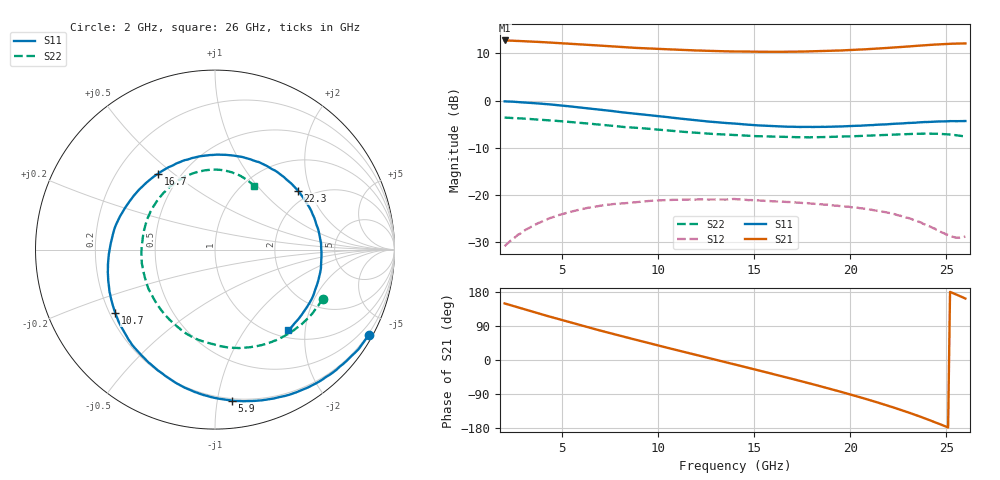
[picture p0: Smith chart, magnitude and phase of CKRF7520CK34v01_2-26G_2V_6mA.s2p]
! CHUO DENSHI KOGYO Co.,Ltd.
! 1. March 2016
! CKRF7520CK34
! N-channel HJ-FET
! Vds = 2 V Id = 6 mA
# Hz S  MA  R 50
!  f  S11  S21  S12  S22
!  Hz  MAG  ANG  MAG  ANG  MAG  ANG  MAG  ANG
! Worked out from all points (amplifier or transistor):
!   241 points, 2 GHz to 26 GHz, reference 50 ohm
!   highest |S21| = 12.7 dB at 2 GHz (marker M1)
!   |S21| within 3 dB of that: start of sweep to end of sweep
!   unconditionally stable (mu >= 1): 14.56 GHz to end of sweep
!   at 6 GHz: K = 0.47, MSG = 17.5 dB, |S12| = -23.0 dB
!   at 14 GHz: K = 0.96, MSG = 15.6 dB, |S12| = -20.9 dB
!   at 26 GHz: K = 1.72, MAG = 15.5 dB, |S12| = -28.8 dB
!   S11 on the Smith chart (normalised r, x): 2 GHz: 0.16, -3.84; 5.9 GHz: 0.19, -1.10; 10.7 GHz: 0.22, -0.28; 16.7 GHz: 0.38, +0.44; 22.3 GHz: 1.72, +1.66; 26 GHz: 1.14, -1.62
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2e9  0.9804 -29.2  4.329 149.3  0.02863 67.6  0.6592 -24.5
3e9  0.9529 -43.3  4.248 134.2  0.04155 56.8  0.6435 -36.6
4e9  0.9217 -57.5  4.152 119.5  0.05287 46.0  0.6236 -48.0
4.9e9  0.8871 -69.9  4.055 106.6  0.06186 37.1  0.6043 -58.2
5.9e9  0.8465 -83.6  3.939 92.5  0.06966 27.6  0.5806 -69.0
6e9  0.8418 -84.9  3.926 91.1  0.0706 26.7  0.5784 -70.0
7.9e9  0.7598 -110.3  3.708 65.3  0.08066 9.5  0.5314 -89.5
1e10  0.6827 -137.9  3.525 38.4  0.0874 -6.3  0.4917 -110.1
1.07e10  0.6589 -147.4  3.473 29.4  0.0885 -11.5  0.4765 -116.8
1.24e10  0.6045 -170.6  3.37 8.0  0.08943 -23.3  0.4492 -132.8
1.4e10  0.5701 166.8  3.308 -11.9  0.09041 -34.0  0.431 -148.2
1.53e10  0.5439 147.8  3.287 -28.4  0.08704 -43.0  0.4181 -161.3
1.67e10  0.5281 126.8  3.29 -46.2  0.08414 -51.3  0.4109 -175.8
1.8e10  0.5243 107.0  3.32 -63.3  0.08084 -59.7  0.4083 170.4
2.01e10  0.5379 73.5  3.431 -92.3  0.07388 -74.6  0.418 146.2
2.11e10  0.5486 56.7  3.521 -107.1  0.06975 -83.1  0.4256 133.7
2.2e10  0.5625 40.7  3.614 -121.1  0.06459 -92.2  0.4337 122.0
2.23e10  0.5672 35.2  3.647 -126.0  0.06261 -96.0  0.4357 117.9
2.34e10  0.5819 13.8  3.788 -145.0  0.05373 -113.1  0.4439 102.0
2.44e10  0.5967 -7.9  3.914 -163.8  0.04399 -136.1  0.4453 86.4
2.52e10  0.605 -27.0  3.991 179.8  0.03669 -165.3  0.4363 72.8
2.6e10  0.6063 -47.9  4.028 162.2  0.03623 153.7  0.416 58.2
